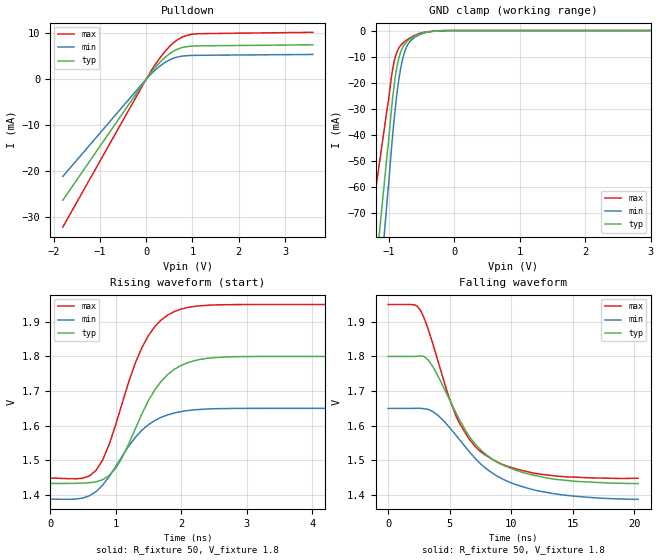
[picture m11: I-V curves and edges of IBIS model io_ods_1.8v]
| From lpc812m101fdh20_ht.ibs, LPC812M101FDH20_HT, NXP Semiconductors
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[Model]   io_ods_1.8v
Model_type I/O_open_drain
Vinl=5.400E-01
Vinh=1.260E+00
Vref=1.800E+00
Rref=1.000E+03
Cref=2.000E-11
Vmeas=9.000E-01
C_comp   8.440E-13   8.280E-13   8.600E-13
[Voltage Range]   1.800E+00   1.650E+00   1.950E+00
[POWER Clamp Reference]   1.800E+00   1.650E+00   1.950E+00
[GND Clamp Reference]   0.000E+00   0.000E+00   0.000E+00
[Pullup Reference]   1.800E+00   1.650E+00   1.950E+00
[Pulldown Reference]   0.000E+00   0.000E+00   0.000E+00
[Temperature Range]   25   105   -40
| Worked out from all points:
|   slope of the pulldown table from 0 to 0.27 V, typ, clamps not added: 80.1 ohm
|   GND clamp passes 1 mA (typ) near -0.49 V on its own axis
|   rising waveform, R_fixture 50, V_fixture 1.8: 20-80 % time 595ps typ, 618ps min, 564ps max; typ from 1.43 V to 1.8 V
|   falling waveform, R_fixture 50, V_fixture 1.8: 20-80 % time 4.05ns typ, 4.73ns min, 3.36ns max; typ from 1.8 V to 1.43 V
[GND Clamp]
-1.8V     -244.7mA   -294.7mA   -167mA
-1.02V    -46.52mA   -64.09mA   -29.35mA
-940mV    -25.93mA   -40.25mA   -14.92mA
-900mV    -17.84mA   -29.88mA   -10.21mA
-860mV    -12.13mA   -21.41mA   -7.428mA
-820mV    -8.42mA    -14.88mA   -5.782mA
-780mV    -6.161mA   -10.21mA   -4.745mA
-740mV    -4.723mA   -7.073mA   -3.919mA
-680mV    -3.339mA   -4.344mA   -2.881mA
-500mV    -1.101mA   -1.317mA   -892.5uA
-240mV    -116.5uA   -126.1uA   -97.57uA
3.6V      0A         0A         0A
[Pulldown]
-1.8V     -26.45mA   -21.25mA   -32.33mA
0V        0A         0A         0A
140mV     1.894mA    1.494mA    2.352mA
320mV     3.921mA    3.039mA    4.945mA
500mV     5.53mA     4.194mA    7.104mA
600mV     6.19mA     4.629mA    8.047mA
740mV     6.8mA      4.988mA    8.997mA
880mV     7.124mA    5.147mA    9.584mA
1.14V     7.298mA    5.229mA    9.953mA
3.6V      7.517mA    5.412mA    10.25mA
[Rising Waveform]
R_fixture = 50
V_fixture = 1.8
V_fixture_min = 1.65
V_fixture_max = 1.95
0s        1.433V     1.388V     1.448V
500ps     1.434V     1.391V     1.448V
700ps     1.438V     1.41V      1.471V
800ps     1.444V     1.428V     1.501V
1ns       1.477V     1.482V     1.603V
1.4ns     1.634V     1.587V     1.826V
1.6ns     1.705V     1.615V     1.887V
1.9ns     1.763V     1.637V     1.93V
2.6ns     1.798V     1.649V     1.949V
5.7ns     1.8V       1.65V      1.95V
[Falling Waveform]
R_fixture = 50
V_fixture = 1.8
V_fixture_min = 1.65
V_fixture_max = 1.95
0s        1.8V       1.65V      1.95V
2.1ns     1.8V       1.65V      1.949V
2.6ns     1.801V     1.65V      1.935V
3.6ns     1.773V     1.642V     1.84V
5.5ns     1.638V     1.573V     1.629V
6.6ns     1.569V     1.525V     1.561V
7.8ns     1.521V     1.481V     1.518V
9.4ns     1.485V     1.444V     1.487V
12.1ns    1.455V     1.413V     1.462V
20.3ns    1.433V     1.388V     1.448V
[Ramp]
dV/dt_r   2.2020E-01/5.9240E-10   1.5747E-01/6.1240E-10   3.0112E-01/5.6020E-10
dV/dt_f   2.2020E-01/4.0369E-09   1.5747E-01/4.7266E-09   3.0112E-01/3.3543E-09
R_load = 50
